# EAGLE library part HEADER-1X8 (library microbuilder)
PIN HEADER
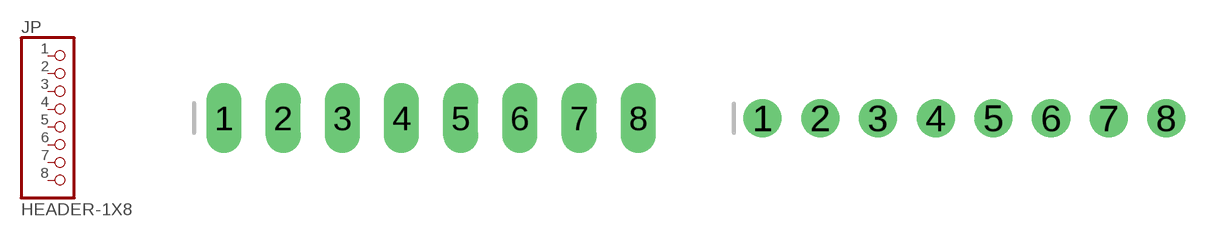
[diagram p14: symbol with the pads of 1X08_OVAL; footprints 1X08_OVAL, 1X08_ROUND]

Designator prefix JP

## HEADER-1X8  [1X08_OVAL]
1  1  pas
2  2  pas
3  3  pas
4  4  pas
5  5  pas
6  6  pas
7  7  pas
8  8  pas

## HEADER-1X8ROUND  [1X08_ROUND]
Pads as for 1X08_OVAL

## HEADER-1X876MIL  [1X08_ROUND_76]
Pads as for 1X08_OVAL

## HEADER-1X870MIL  [1X08_ROUND_70]
Pads as for 1X08_OVAL

## Footprint 1X08_OVAL (pad centres in mm)
PIN HEADER
drill 1 long: 1 -8.89,0; 2 -6.35,0; 3 -3.81,0; 4 -1.27,0; 5 1.27,0; 6 3.81,0; 7 6.35,0; 8 8.89,0

## Footprint 1X08_ROUND (pad centres in mm)
drill 1 pad 1.676: 1 -8.89,0; 2 -6.35,0; 3 -3.81,0; 4 -1.27,0; 5 1.27,0; 6 3.81,0; 7 6.35,0; 8 8.89,0

## Footprint 1X08_ROUND_76 (pad centres in mm)
drill 1 pad 1.93: 1 -8.89,0; 2 -6.35,0; 3 -3.81,0; 4 -1.27,0; 5 1.27,0; 6 3.81,0; 7 6.35,0; 8 8.89,0

## Footprint 1X08_ROUND_70 (pad centres in mm)
drill 1 pad 1.778: 1 -8.89,0; 2 -6.35,0; 3 -3.81,0; 4 -1.27,0; 5 1.27,0; 6 3.81,0; 7 6.35,0; 8 8.89,0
